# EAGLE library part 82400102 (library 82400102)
TVS Diode Array WE-TVS SOT23-6L; 5Vdc; 2pF; 2Channel + VDD; Marking: .W00XY Source: Datasheet
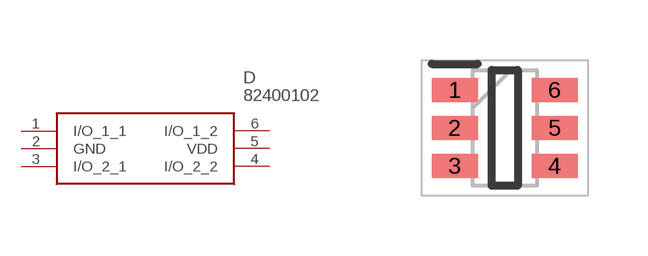
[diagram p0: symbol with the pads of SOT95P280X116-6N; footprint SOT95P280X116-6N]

Designator prefix D

## 82400102 (Description: TVS Diode Array WE-TVS SOT23-6L; 5Vdc; 2pF; 2Channel + VDD; Marking: .W00XY; Height: 1.16mm; Manufacturer_Name: Wurth Elektronik; Manufacturer_Part_Number: 82400102; Mouser_Part_Number: 710-82400102; Mouser_Price-Stock: https://www.mouser.co.uk/ProductDetail/Wurth-Elektronik/82400102?qs=Wn16VcyqZWq4x2NXBP4V%252Bw%3D%3D)  [SOT95P280X116-6N]
1  I/O_1_1
2  GND
3  I/O_2_1
4  I/O_2_2
5  VDD
6  I/O_1_2

## Footprint SOT95P280X116-6N (pad centres in mm)
SOT23-6L_2020
smd 1.15 x 0.6: 1 -1.25,0.95; 2 -1.25,0; 3 -1.25,-0.95; 4 1.25,-0.95; 5 1.25,0; 6 1.25,0.95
